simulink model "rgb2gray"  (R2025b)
settings: Solver=VariableStepDiscrete  StartTime=0.0  StopTime=20  RelTol=1e-3  EnableMultiTasking=on
undefined symbols (not defined in the file or in its folder): Addsub_config, AXI4, C, CMult_config, code, Constant_config, Convert_config, Evaluation, ffva1156, gateway_in_config, gateway_out_config, hex2dec, HLS, KCU105, Kintex, Lite, netlist, Platform, Reinterpret_config, sysgen, UltraScale, xcku040
libraries: hdlBasic x13, vmcUtilities x1

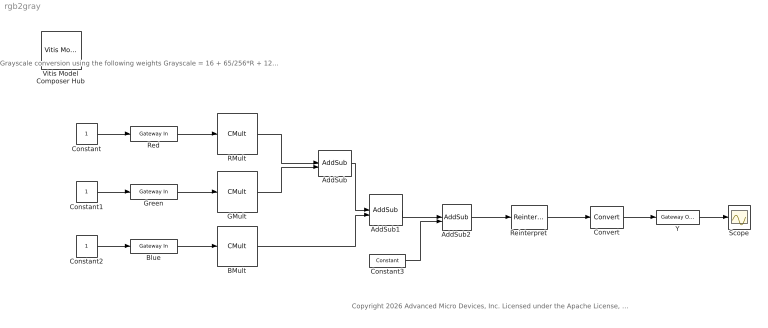
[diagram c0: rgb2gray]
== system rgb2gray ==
  note: Grayscale conversion using the following weights Grayscale = 16 + 65/256*R + 129/256*G + 25/256*B
  note: Copyright 2026 Advanced Micro Devices, Inc. Licensed under the Apache License, Version 2.0 (the "License"); you may not use this file except in compliance with the License. You may obtain a copy of the License at http://www.apache.org/licenses/LICENSE-2.0 Unless required by applicable law or agreed to in writing, software distributed under the License is distributed on an "AS IS" BASIS, WITHOUT WARRANTIES OR CONDITIONS OF ANY KIND, either express or implied. See the License for the specific language governing permissions and limitations under the License.
  AddSub : hdlBasic/AddSub  mode=Addition  use_carryin=off  use_carryout=off  en=off  latency=1  precision=Full  arith_type=Unsigned  n_bits=8  bin_pt=2  quantization=Truncate  overflow=Wrap  use_behavioral_HDL=on  hw_selection=Fabric  pipelined=off  use_rpm=on  XmcBlockStatus=1  maskContainerNames=tabcontainer1  block_type=addsub  block_config=sysgen:Addsub_config
  AddSub1 : hdlBasic/AddSub  mode=Addition  use_carryin=off  use_carryout=off  en=off  latency=0  precision=Full  arith_type=Unsigned  n_bits=8  bin_pt=2  quantization=Truncate  overflow=Wrap  use_behavioral_HDL=on  hw_selection=Fabric  pipelined=off  use_rpm=on  XmcBlockStatus=1  maskContainerNames=tabcontainer1  block_type=addsub  block_config=sysgen:Addsub_config
  AddSub2 : hdlBasic/AddSub  mode=Addition  use_carryin=off  use_carryout=off  en=off  latency=1  precision=Full  arith_type=Unsigned  n_bits=8  bin_pt=2  quantization=Truncate  overflow=Wrap  use_behavioral_HDL=on  hw_selection=Fabric  pipelined=off  use_rpm=on  XmcBlockStatus=1  maskContainerNames=tabcontainer1  block_type=addsub  block_config=sysgen:Addsub_config
  BMult : hdlBasic/CMult  const=25  gui_display_data_type=Fixed-point  const_n_bits=8  const_bin_pt=0  float_type=Single  exp_bits=8  fraction_bits=24  en=off  latency=1  precision=Full  arith_type="Signed  (2's comp)"  n_bits=8  bin_pt=6  quantization="Round  (unbiased: +/- Inf)"  overflow=Wrap  use_behavioral_HDL=off  mem_type=Distributed RAM  pipeline=off  use_rpm=on  placement_style=Rectangular Shape  XmcBlockStatus=1  maskContainerNames=tabcontainer1  block_type=cmult  block_config=sysgen:CMult_config
  Blue : hdlBasic/Gateway In  gui_display_data_type=Fixed-point  arith_type=Unsigned  n_bits=8  bin_pt=0  preci_type=Single  exp_width=8  frac_width=24  rows=1  columns=1  quantization="Round  (unbiased: +/- Inf)"  overflow=Saturate  period=1  UseAsADC=off  ADCChannel='1'  interface=AXI4-Lite  automatic_assignment=on  address_offset=hex2dec('00')  intf_name=''  intf_description='Blue'  default_value=0  timing_constraint=None  locs_specified=off  LOCs={}  io_standard={}  inherit_from_input=off  hdl_port=on  XmcBlockStatus=1  maskContainerNames=group4  block_type=gatewayin  block_config=sysgen:gateway_in_config  block_width_w=590  block_height_w=620  block_width=640  block_height=850
  Constant : Constant
  Constant1 : Constant
  Constant2 : Constant
  Constant3 : hdlBasic/Constant  const=16*256  gui_display_data_type=Fixed-point  arith_type=Unsigned  n_bits=16  bin_pt=0  preci_type=Single  exp_width=8  frac_width=24  explicit_period=off  period=1  XmcBlockStatus=1  maskContainerNames=tabcontainer1  block_type=constant  block_config=sysgen:Constant_config
  Convert : hdlBasic/Convert  gui_display_data_type=Fixed-point  arith_type=Unsigned  n_bits=8  bin_pt=0  float_type=Single  exp_bits=8  fraction_bits=24  quantization="Round  (unbiased: Even Values)"  overflow=Saturate  en=off  latency=0  pipeline=off  XmcBlockStatus=1  maskContainerNames=group2  block_type=convert  block_config=sysgen:Convert_config  block_width=595  block_height=885
  GMult : hdlBasic/CMult  const=129  gui_display_data_type=Fixed-point  const_n_bits=8  const_bin_pt=0  float_type=Single  exp_bits=8  fraction_bits=24  en=off  latency=0  precision=Full  arith_type="Signed  (2's comp)"  n_bits=8  bin_pt=6  quantization="Round  (unbiased: +/- Inf)"  overflow=Wrap  use_behavioral_HDL=off  mem_type=Distributed RAM  pipeline=off  use_rpm=on  placement_style=Rectangular Shape  XmcBlockStatus=1  maskContainerNames=tabcontainer1  block_type=cmult  block_config=sysgen:CMult_config
  Green : hdlBasic/Gateway In  gui_display_data_type=Fixed-point  arith_type=Unsigned  n_bits=8  bin_pt=0  preci_type=Single  exp_width=8  frac_width=24  rows=1  columns=1  quantization="Round  (unbiased: +/- Inf)"  overflow=Saturate  period=1  UseAsADC=off  ADCChannel='1'  interface=AXI4-Lite  automatic_assignment=on  address_offset=hex2dec('02')  intf_name=''  intf_description='Green'  default_value=0  timing_constraint=None  locs_specified=off  LOCs={}  io_standard={}  inherit_from_input=off  hdl_port=on  XmcBlockStatus=1  maskContainerNames=group4  block_type=gatewayin  block_config=sysgen:gateway_in_config  block_width_w=590  block_height_w=620  block_width=640  block_height=850
  RMult : hdlBasic/CMult  const=65  gui_display_data_type=Fixed-point  const_n_bits=8  const_bin_pt=0  float_type=Single  exp_bits=8  fraction_bits=24  en=off  latency=0  precision=Full  arith_type="Signed  (2's comp)"  n_bits=8  bin_pt=6  quantization="Round  (unbiased: +/- Inf)"  overflow=Wrap  use_behavioral_HDL=off  mem_type=Distributed RAM  pipeline=off  use_rpm=on  placement_style=Rectangular Shape  XmcBlockStatus=1  maskContainerNames=tabcontainer1  block_type=cmult  block_config=sysgen:CMult_config
  Red : hdlBasic/Gateway In  gui_display_data_type=Fixed-point  arith_type=Unsigned  n_bits=8  bin_pt=0  preci_type=Single  exp_width=8  frac_width=24  rows=1  columns=1  quantization="Round  (unbiased: +/- Inf)"  overflow=Saturate  period=1  UseAsADC=off  ADCChannel='1'  interface=AXI4-Lite  automatic_assignment=on  address_offset=hex2dec('00')  intf_name=''  intf_description='Red'  default_value=0  timing_constraint=None  locs_specified=off  LOCs={}  io_standard={}  inherit_from_input=off  hdl_port=on  XmcBlockStatus=1  maskContainerNames=group4  block_type=gatewayin  block_config=sysgen:gateway_in_config  block_width_w=590  block_height_w=620  block_width=640  block_height=850
  Reinterpret : hdlBasic/Reinterpret  force_arith_type=off  arith_type=Unsigned  force_bin_pt=on  bin_pt=8  XmcBlockStatus=1  maskContainerNames=group1  block_type=reinterpret  block_config=sysgen:Reinterpret_config
  Scope : Scope
  Vitis Model Composer Hub : vmcUtilities/Vitis Model Composer Hub  Tag=genX  CodeGeneration=off  SubsystemName=<enter or select subsystem name>  StartColumn=1  NumberOfColumns=1  TargetDirectory=./code  exportDesign=off  analyzeDesign=off  validateDesignOnHw=off  ExportType=HLS C++ code  IpVendor=xilinx.com  IpLibrary=hls  IpVersion=1.0  IpHWLanguage=Verilog  AieCompilerOptions={}  AieSimulatorOptions={}  CreateTestbench=off  TestbenchStackSize=10  RunRtlSim=off  RunCSim=off  RunAieSim=off  AieSimTimeout=50000  RunAieSimProfiling=off  LaunchVitisAnalyzer=off  PlotOutput=off  RunX86Sim=off  X86SimTimeout=10  GenHwImage=off  GenLibadfXo=off  GenHwValidationCode=off  PlatformType=Not Specified  HwSystemType=Baremetal  HwValidationTarget=hw  ProjDevice=Kintex-UltraScale KCU105 Evaluation Platform (xcku040-ffva1156-2-e)  ProjDevicePart=xcku040-ffva1156-2-e  SamplePeriod=-1  ClockFrequency=200  DataPathParallelism=1  xilinxfamily=kintexu  part=xcku040  speed=-2-e  package=ffva1156  directory=./netlist  testbench=off  incr_netlist=off  synthesis_tool=Vivado  clock_wrapper=Clock Enables  dbl_ovrd=According to Block Masks  dcm_input_clock_period=10  sysclk_period=10  simulink_period=1  eval_field=0  LogFileName=''  NThreads=4
  Y : hdlBasic/Gateway Out  inherit_from_input=off  bool_to_boolean=off  hdl_port=on  rows=1  columns=1  UseAsDAC=off  DACChannel='1'  interface=AXI4-Lite  automatic_assignment=on  address_offset=hex2dec('00')  intf_name=''  intf_description='Luminance'  timing_constraint=None  locs_specified=off  LOCs={}  io_standard={}  XmcBlockStatus=1  maskContainerNames=group4  block_type=gatewayout  block_config=sysgen:gateway_out_config  block_width_w=590  block_height_w=620  block_width=620  block_height=750
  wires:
  AddSub/1 -> AddSub1/1
  GMult/1 -> AddSub/2
  Blue/1 -> BMult/1
  Green/1 -> GMult/1
  Red/1 -> RMult/1
  BMult/1 -> AddSub1/2
  AddSub1/1 -> AddSub2/1
  Constant/1 -> Red/1
  Constant1/1 -> Green/1
  Constant2/1 -> Blue/1
  Y/1 -> Scope/1
  Constant3/1 -> AddSub2/2
  AddSub2/1 -> Reinterpret/1
  Reinterpret/1 -> Convert/1
  Convert/1 -> Y/1
  RMult/1 -> AddSub/1
